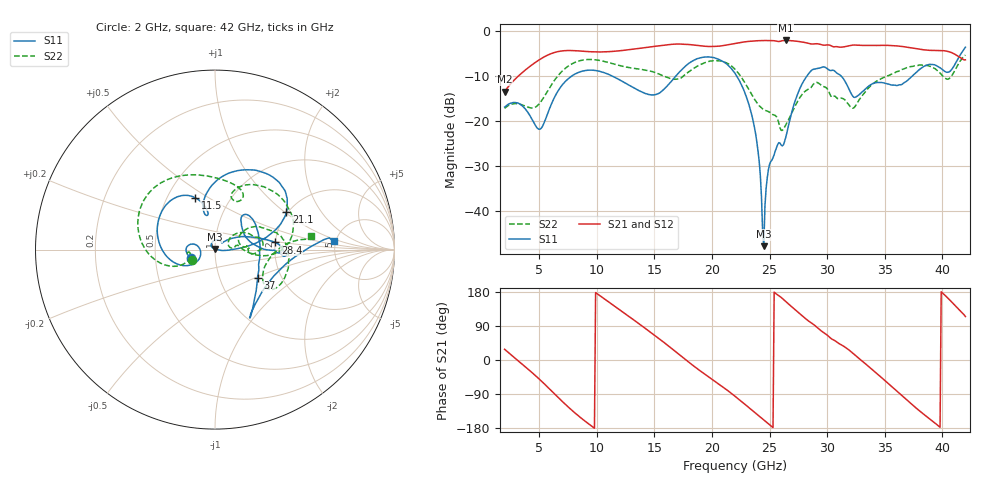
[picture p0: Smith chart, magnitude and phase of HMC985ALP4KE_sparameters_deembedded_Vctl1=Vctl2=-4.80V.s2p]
!s2p File: Measurements: S11, S21, S12, S22
# GHz S dB R 50.0
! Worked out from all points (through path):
!   401 points, 2 GHz to 42 GHz, reference 50 ohm
!   highest |S21| = -2.06 dB at 26.4 GHz (marker M1); lowest = -13.4 dB at 2 GHz (marker M2)
!   lowest |S11| = -47.8 dB at 24.5 GHz (marker M3), VSWR 1.01, Z = 49.8 + j0.376 ohm
!   |S11| at or under -10 dB: start of sweep to 7.814 GHz; 22.15 GHz to 28.23 GHz (6.08 GHz wide, 24.1 % of centre); 31.22 GHz to 37.38 GHz (6.153 GHz wide, 17.9 % of centre)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
!   |S22| runs from -22.1 to -5.3 dB; largest |S21 - S12| = 0.00092
!   S11 on the Smith chart (normalised r, x): 2 GHz: 0.76, -0.07; 11.5 GHz: 0.69, +0.44; 21.1 GHz: 1.97, +1.02; 28.4 GHz: 2.00, +0.18; 37 GHz: 1.51, -0.52; 42 GHz: 4.82, +0.78
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2  -16.86 -161.7  -13.43 28.2  -13.44 28.2  -17.17 -155.6
5  -21.81 -172.7  -6.37 -50.1  -6.38 -50.1  -16.16 -159.8
6.3  -14.85 -150.3  -4.76 -88.4  -4.76 -88.4  -11.02 -161.6
8.7  -8.92 150.3  -4.44 -154.6  -4.44 -154.6  -6.46 151.2
11.5  -10.17 111.1  -4.47 143.1  -4.47 143.1  -7.31 105.0
13.6  -13.13 101.2  -3.85 97.1  -3.85 97.1  -8.40 75.6
15.4  -13.81 105.9  -3.25 56.4  -3.25 56.4  -9.51 62.0
17.9  -7.32 80.2  -2.94 -3.6  -2.94 -3.6  -9.19 72.0
21.1  -6.97 27.5  -3.14 -74.5  -3.14 -74.4  -6.87 15.9
22  -9.36 17.0  -2.71 -95.7  -2.71 -95.6  -8.46 0.5
23.6  -20.27 0.2  -2.18 -135.4  -2.17 -135.3  -14.74 -4.5
24.5  -47.81 112.0  -2.08 -158.0  -2.08 -158.0  -17.41 8.1
25  -29.61 131.8  -2.10 -170.8  -2.10 -170.7  -18.00 11.0
26.4  -23.66 41.5  -2.06 154.5  -2.06 154.5  -20.92 32.8
28.4  -9.42 6.8  -2.71 102.5  -2.71 102.6  -12.86 18.2
28.7  -8.59 1.9  -2.85 96.3  -2.86 96.3  -12.18 16.2
30.7  -8.96 -3.1  -3.44 50.4  -3.45 50.5  -14.48 2.0
32.5  -14.62 31.8  -3.10 10.7  -3.09 10.7  -16.45 27.6
35.4  -11.81 19.1  -3.17 -64.8  -3.16 -64.8  -9.79 19.3
37  -10.88 -33.8  -3.58 -107.9  -3.58 -107.9  -8.06 4.9
39.8  -8.12 -57.4  -4.29 -177.5  -4.29 -177.5  -9.30 -35.9
42  -3.56 3.9  -6.36 114.8  -6.37 114.8  -5.31 8.2
